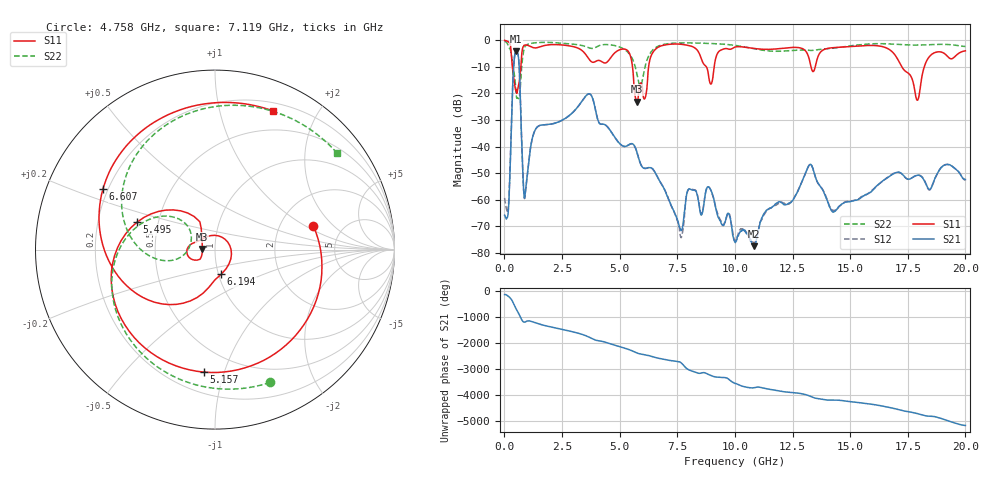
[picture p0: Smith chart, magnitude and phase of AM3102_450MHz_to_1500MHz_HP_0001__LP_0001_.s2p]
!Agilent Technologies,E8364B,MY43040894,A.07.50.67
!Agilent E8364B: A.07.50.67
!Date: Thursday, January 11, 2018 05:19:49
!Correction: S11(Full 2 Port(1,2))
!S21(Full 2 Port(1,2))
!S12(Full 2 Port(1,2))
!S22(Full 2 Port(1,2))
!S2P File: Measurements: S11, S21, S12, S22:
# Hz S  dB  R 50
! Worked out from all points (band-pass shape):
!   1601 points, 10 MHz to 20 GHz, reference 50 ohm
!   highest |S21| = -4.09 dB at 509.8 MHz (marker M1); lowest = -77.4 dB at 10.83 GHz (marker M2)
!   |S21| within 3 dB of the highest: 429.1 MHz to 619.1 MHz (190 MHz wide, 36.3 % of centre)
!   lowest |S11| = -23.0 dB at 5.745 GHz (marker M3), VSWR 1.15, Z = 43.4 + j0.336 ohm
!   |S11| at or under -10 dB: 347.1 MHz to 714.5 MHz (367.4 MHz wide, 69.2 % of centre); 5.559 GHz to 6.257 GHz (697.8 MHz wide, 11.8 % of centre); 17.24 GHz to 18.21 GHz (971.9 MHz wide, 5.48 % of centre)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
!   |S22| runs from -21.9 to -0.4 dB; largest |S21 - S12| = 0.0018
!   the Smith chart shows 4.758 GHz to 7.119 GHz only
!   S11 on the Smith chart (normalised r, x): 4.758 GHz: 3.09, +1.18; 5.157 GHz: 0.33, -0.86; 5.495 GHz: 0.38, +0.15; 6.194 GHz: 1.03, -0.29; 6.607 GHz: 0.18, +0.25; 7.119 GHz: 0.28, +1.46
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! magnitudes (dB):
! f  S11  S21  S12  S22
! 10 MHz  -0.1  -65.8  -59.3  -0.4
! 172.4 MHz  -0.6  -64.1  -62.5  -2.1
! 509.8 MHz  -18.5  -4.1  -4.1  -20.4
! 897.1 MHz  -1.8  -58.2  -58.4  -2.3
! 1.384 GHz  -2.8  -33.0  -33.0  -0.9
! 3.346 GHz  -3.7  -23.1  -23.1  -1.9
! 4.758 GHz  -5.0  -36.1  -36.1  -1.9
! 5.157 GHz  -3.3  -39.8  -39.8  -3.1
! 5.495 GHz  -6.7  -38.9  -38.9  -6.0
! 5.745 GHz  -23.0  -42.0  -41.9  -12.5
! 6.194 GHz  -17.0  -48.0  -48.0  -7.3
! 6.607 GHz  -3.0  -50.9  -50.9  -2.5
! 6.682 GHz  -2.5  -52.1  -52.1  -2.2
! 7.119 GHz  -1.5  -59.7  -59.7  -1.2
! 8.881 GHz  -14.6  -55.3  -55.3  -1.2
! 10.01 GHz  -2.6  -75.9  -75.4  -1.9
! 10.83 GHz  -3.1  -77.4  -76.3  -3.2
! 13.34 GHz  -11.1  -47.3  -47.3  -3.8
! 14.28 GHz  -2.8  -64.6  -64.0  -2.9
! 16.68 GHz  -3.3  -51.3  -51.3  -1.3
! 17.91 GHz  -22.5  -50.8  -50.8  -1.8
! 20 GHz  -4.0  -52.4  -52.6  -2.3
